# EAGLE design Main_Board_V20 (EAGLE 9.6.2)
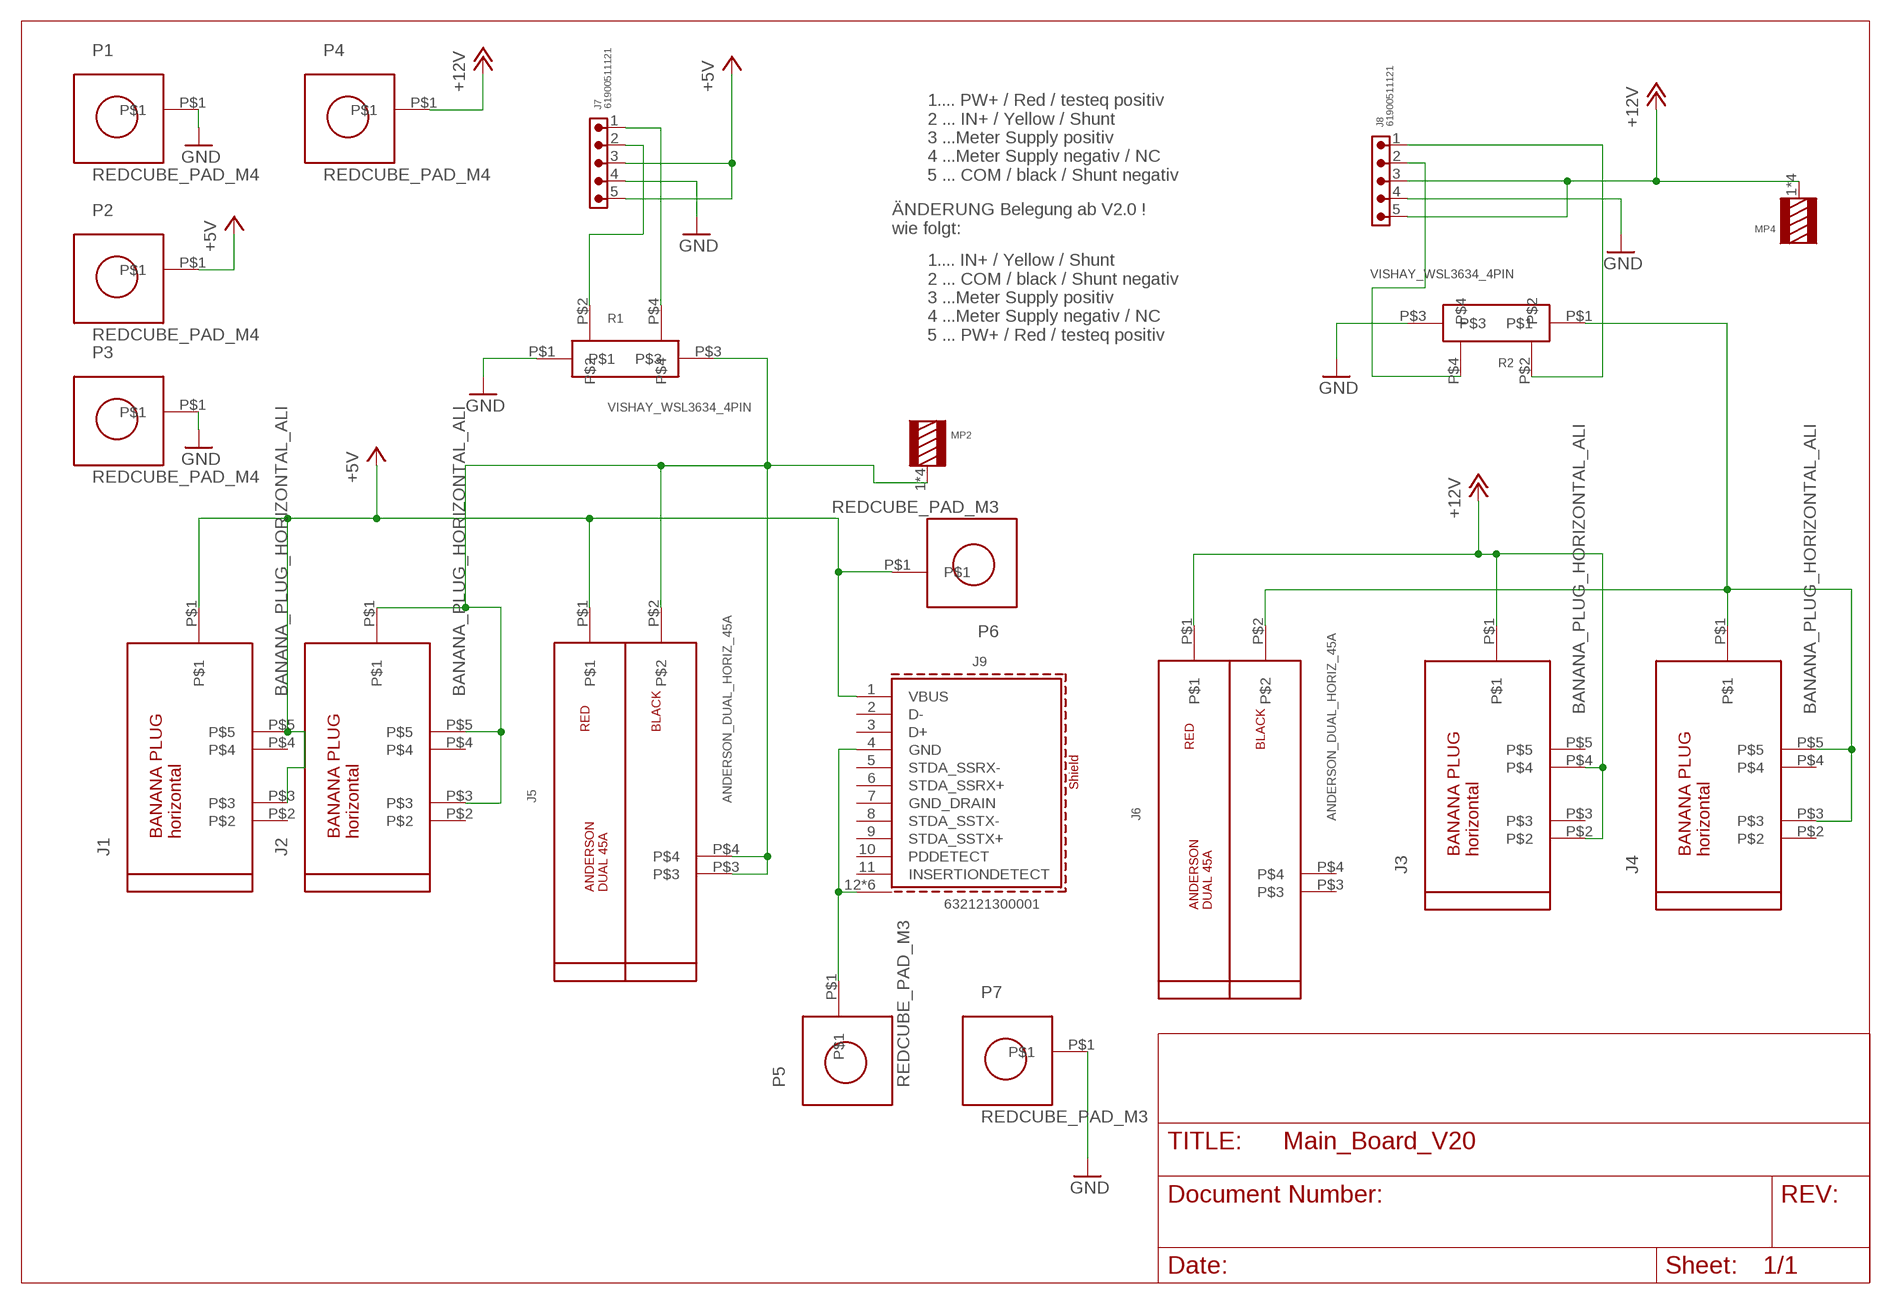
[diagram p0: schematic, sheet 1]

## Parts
J1  BANANA_PLUG_HORIZONTAL_ALI  [BANANA_PLUG_HORIZONTAL_ALI]
J2  BANANA_PLUG_HORIZONTAL_ALI  [BANANA_PLUG_HORIZONTAL_ALI]
J3  BANANA_PLUG_HORIZONTAL_ALI  [BANANA_PLUG_HORIZONTAL_ALI]
J4  BANANA_PLUG_HORIZONTAL_ALI  [BANANA_PLUG_HORIZONTAL_ALI]
J5  ANDERSON_DUAL_HORIZ_45A  [ANDERSON_DUAL_HORIZ_45A]
J6  ANDERSON_DUAL_HORIZ_45A  [ANDERSON_DUAL_HORIZ_45A]
J7  61900511121  61900511121  [61900511121]
J8  61900511121  61900511121  [61900511121]
J9  632121300001  [632121300001_MILLING_LINES]
MP2  WP-THRBU_THROUGH-HOLE_74650073R  [WP-THRBU_74650073]
MP4  WP-THRBU_THROUGH-HOLE_74650073R  [WP-THRBU_74650073]
P1  REDCUBE_PAD_M4  [REDCUBE_PAD_M4]
P2  REDCUBE_PAD_M4  [REDCUBE_PAD_M4]
P3  REDCUBE_PAD_M4  [REDCUBE_PAD_M4]
P4  REDCUBE_PAD_M4  [REDCUBE_PAD_M4]
P5  REDCUBE_PAD_M3  [REDCUBE_PAD_M3]
P6  REDCUBE_PAD_M3  [REDCUBE_PAD_M3]
P7  REDCUBE_PAD_M3  [REDCUBE_PAD_M3]
R1  VISHAY_WSL3634_4PIN  [VISHAY_WSL3637_4PIN]
R2  VISHAY_WSL3634_4PIN  [VISHAY_WSL3637_4PIN]

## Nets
+5V [Versorgung]: J1.P$1 J1.P$3 J1.P$5 J5.P$1 J7.3 J7.5 J9.1(VBUS) P2.P$1 P6.P$1
+12V [Versorgung]: J3.P$1 J3.P$2 J3.P$4 J6.P$1 J8.3 J8.5 MP4.1 MP4.2 MP4.3 MP4.4 P4.P$1
GND [Versorgung]: J7.4 J8.4 P1.P$1 P3.P$1 P7.P$1 R1.P$1 R2.P$3
N$2 [Versorgung]: J4.P$1 J4.P$3 J4.P$5 J6.P$2 R2.P$1
N$3 [Versorgung]: J2.P$1 J2.P$3 J2.P$5 J5.P$2 J5.P$3 J5.P$4 MP2.1 MP2.2 MP2.3 MP2.4 R1.P$3
N$4: J8.1 R2.P$2
N$5: J8.2 R2.P$4
N$6: J7.1 R1.P$4
N$7 [Versorgung]: J9.4(GND) J9.12(SHIELD) J9.13(SHIELD) J9.S1(SHIELD) J9.S2(SHIELD) J9.S3(SHIELD) J9.S4(SHIELD) P5.P$1
N$8: J7.2 R1.P$2
Unconnected: J1.P$2 J1.P$4 J2.P$2 J2.P$4 J3.P$3 J3.P$5 J4.P$2 J4.P$4 J6.P$3 J6.P$4 J9.2(D-) J9.3(D+) J9.5(STDA_SSRX-) J9.6(STDA_SSRX+) J9.7(GND_DRAIN) J9.8(STDA_SSTX-) J9.9(STDA_SSTX+) J9.10(PDDETECT) J9.11(INSERTIONDETECT)

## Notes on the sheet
- 1.... PW+ / Red / testeq positiv
  2 ... IN+ / Yellow / Shunt
  3 ...Meter Supply positiv
  4 ...Meter Supply negativ / NC
  5 ... COM / black / Shunt negativ
- ÄNDERUNG Belegung ab V2.0 !
  wie folgt:
- 1.... IN+ / Yellow / Shunt
  2 ... COM / black / Shunt negativ
  3 ...Meter Supply positiv
  4 ...Meter Supply negativ / NC
  5 ... PW+ / Red / testeq positiv

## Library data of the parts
J1-J4 = Antec-Hood:BANANA_PLUG_HORIZONTAL_ALI
J5 J6 = Antec-Hood:ANDERSON_DUAL_HORIZ_45A
J7 J8 = Eagle_WR-WTB (rev20a):61900511121: WR-WTB 2.54 mm Male Locking Header KIND PROPERTIES: Pitch:2.54 mm Gender:Male MATERIAL PROPERTIES: Insulator Material :PA66 Insulator Flammability Rating:UL94 V-0 Insulator Color:Beige Contact Material:Copper Alloy Contact Plating:Tin Contact Type:Stamped GENERAL INFORMATION Operating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; CONTACT-RESISTANCE: 20mOhm; DATASHEET-URL: https://www.we-online.com/catalog/datasheet/61900511121.pdf; GENDER: Male; L: 12.7mm; MOUNT: THT; PACKAGING: Bag; PART-NUMBER: 61900511121; PCB-CABLE-PANEL: PCB; PINS: 5; PITCH: 2.54mm; TOL-R: max.; TYPE: Vertical; USE-WITH: WR-WTB 2.54 mm Female Terminal Housing; WORKING-VOLTAGE: 250V(AC)
J9 = Antec-Hood:632121300001: WR-COM USB 3.1 Type C Plug Horizontal 0.8 mm Kind Properties Durability:5 000 Mating cycles Quality Class:5 000 Mating cycles Connector Type:USB Gender:Receptacle Type:Horizontal General Information Operating Temperature:-20up to +85 °C Compliance:RoHS Electrical Properties IR 1:5A Working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; APPLICATION: USB 3.1; DATASHEET-URL: https://www.we-online.com/catalog/datasheet/632121300001.pdf; GERDER: Receptacle; INTERFACE-TYPE: Type A; IR1: 5A; MOUNT: THR; PACKAGING: Tray; PART-NUMBER: 632121300001; PINS: 9; TYPE: Horizontal; WORKING-VOLTAGE: 20V(DC)
MP2 MP4 = Eagle_WP-THRBU (rev19a):WP-THRBU_THROUGH-HOLE: WP-THRBU REDCUBE THR internal through-hole thread; DATASHEET-URL: https://katalog.we-online.de/em/datasheet/74650073R.pdf; IR: 50A; PART-NUMBER: 74650073R; PINS: 4; THREAD: M3
P1-P4 = Antec-Hood:REDCUBE_PAD_M4
P5-P7 = Antec-Hood:REDCUBE_PAD_M3
R1 R2 = Antec-Hood:VISHAY_WSL3634_4PIN

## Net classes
1 Versorgung: width 1 mm, drill 0.5 mm, clearance 1 mm

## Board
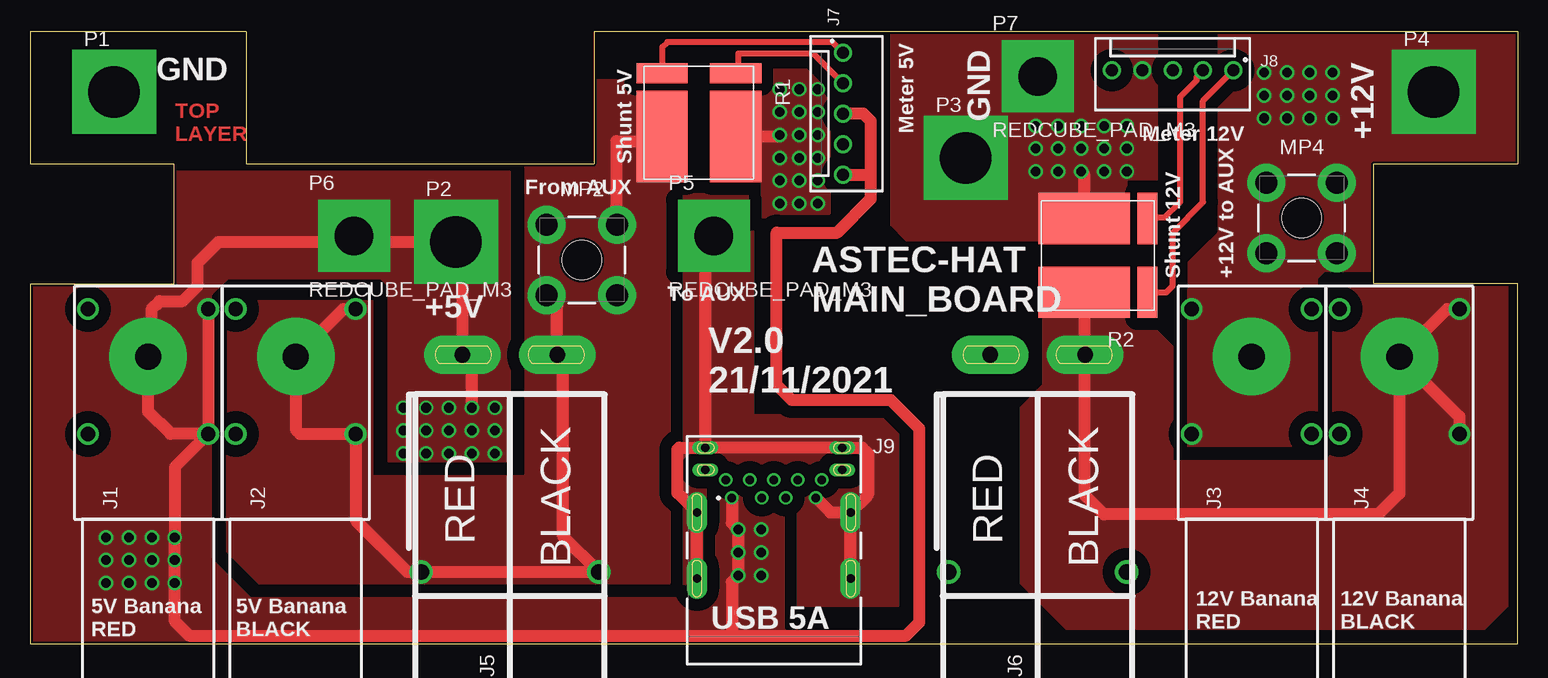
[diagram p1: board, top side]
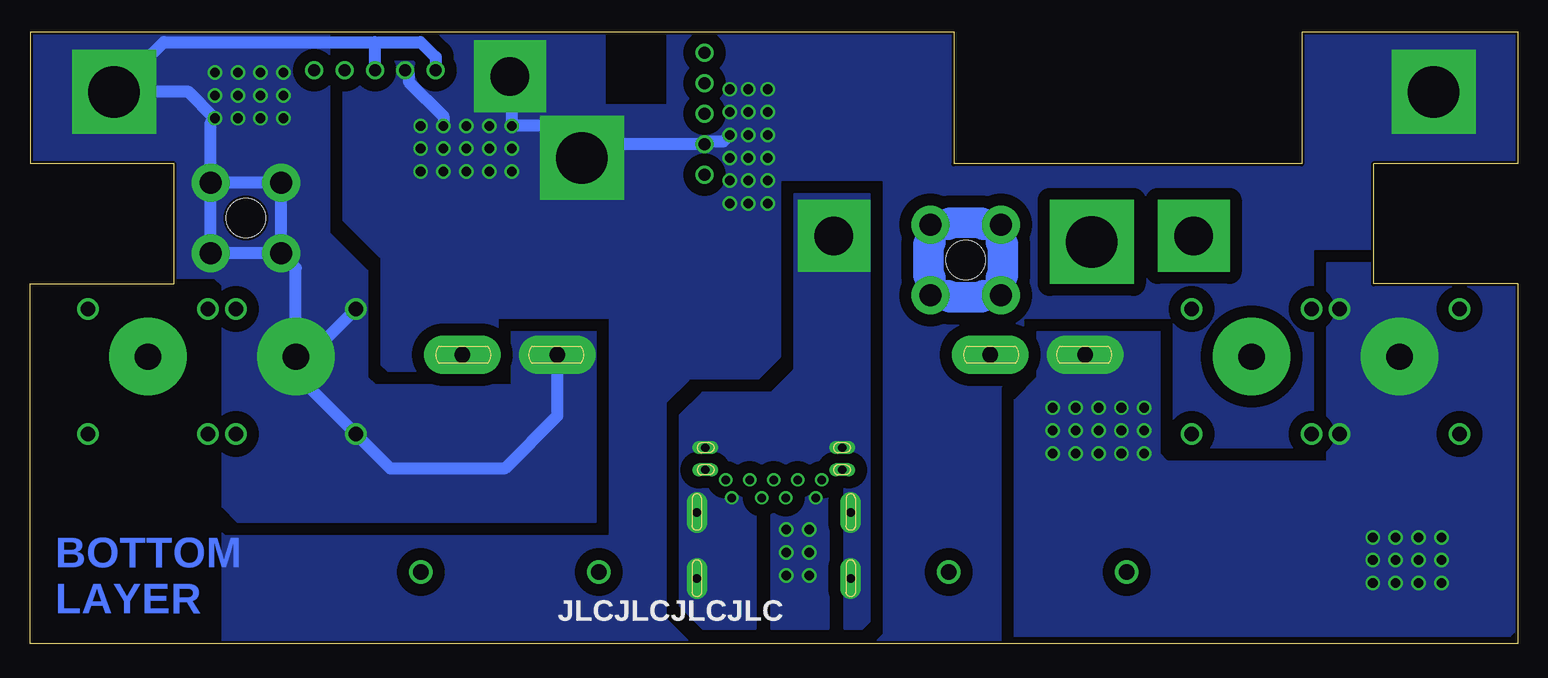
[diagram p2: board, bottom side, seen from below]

Size 124 x 51 mm. Coordinates in mm from the lower left corner, seen from the top.
Outline: 0,0 124,0 124,30 112,30 112,40 124,40 124,51 47,51 47,40 18,40 18,51 0,51 0,40 12,40 12,30 0,30 0,0
Copper layers (1*16): Top 0.035mm / dielectric 1.5mm / Bottom 0.035mm
Design rules "JLCPCB_2alyer": minimum track width 5mil, minimum drill 0.2mm, track to track 5mil, track to pad 0.2mm, pad to pad 0.2mm, via to via 0.2mm, smd to smd 5mil, copper to edge 0.2mm, drill to drill 0.5mm, minimum pad ring 0.13mm, minimum via ring 0.13mm, stop-mask expansion 0.05mm, vias tented up to drill 0mil, thermal gap 10mil
bRestrict: area 71,45 to 76,51

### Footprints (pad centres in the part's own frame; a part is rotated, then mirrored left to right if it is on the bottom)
BANANA_PLUG_HORIZONTAL_ALI = drill 2.2 pad 6.452: P$1 27.94,0 | drill 1.2: P$2 21.5,5; P$3 21.5,-5; P$4 31.9,5; P$5 31.9,-5
ANDERSON_DUAL_HORIZ_45A = drill 1.3 pad 3.2 long: P$1 28.1,3.95; P$2 28.1,-3.95 | drill 1.3: P$3 10,7.4; P$4 10,-7.4
61900511121 = drill 1: 1 5.08,0.3; 2 2.54,0.3; 3 0,0.3; 4 -2.54,0.3; 5 -5.08,0.3
632121300001_MILLING_LINES = drill 0.7 pad 1.1: 1 -3.5,4.425; 2 -1,4.425; 3 1,4.425; 4 3.5,4.425; 5 4,5.925; 6 2,5.925; 7 0,5.925; 8 -2,5.925; 9 -4,5.925 | drill 0.7 pad 1.1 long: 10 -5.7,6.765; 11 5.7,6.765; 12 5.7,8.605; 13 -5.7,8.605 | drill 0.7 pad 1.7 long: S1 -6.4,3.215; S2 6.4,3.215; S3 -6.4,-2.285; S4 6.4,-2.285
WP-THRBU_74650073 = drill 1.85 pad 3.2: 1 -2.935,-2.935; 2 -2.935,2.935; 3 2.935,2.935; 4 2.935,-2.935 | hole 3.3: 0,0
REDCUBE_PAD_M4 = drill 4.3 pad 7 square: P$1 0,0
REDCUBE_PAD_M3 = drill 3.2 pad 6 square: P$1 0,0
VISHAY_WSL3637_4PIN = smd 7.62 x 4.27: P$1 6.1,3.075; P$3 6.1,-3.075 | smd 1.68 x 4.27: P$2 0.84,3.075; P$4 0.84,-3.075

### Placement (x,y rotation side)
J1  9.85,-4 90 top
J2  22.15,-4 90 top
J3  101.85,-4 90 top
J4  114.15,-4 90 top
J5  40,-4 90 top
J6  84,-4 90 top
J7  68.07,44.2 90 top
J8  95.25,47.5 0 top
J9  62,7.75 0 top
MP2  46,32 0 top
MP4  106,35.5 0 top
P1  7,46 0 top
P2  35.5,33.5 0 top
P3  78,40.5 0 top
P4  117,46 0 top
P5  57,34 0 top
P6  27,34 0 top
P7  84,47.3 0 top
R1  55.75,48.39 270 top
R2  93.98,32.38 180 top

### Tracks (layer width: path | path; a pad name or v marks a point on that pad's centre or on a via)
+5V  (via drill 0.8)
  Top 1: 27.3,33.5 15.72,33.5 13.97,31.75 13.97,29.83 12.72,28.57 10.79,28.57 10.16,27.94 10.16,24.25 J1.P$1 9.85,19.36 11.71,17.5 J1.P$3 | 27.3,33.5 P2.P$1 36.05,32.95 J5.P$1 36.83,23.32 v36.83,19.68 | J7.3 69.47,44.2 70.1,43.56 70.1,38.99 | J7.5 69.98,39.12 70.1,38.99 | J1.P$3 12.06,14.71 v12.06,8.89 v12.06,6.99 v12.06,5.08 12.06,1.91 13.27,0.7 58.42,0.7 | J9.1 58.5,10.08 v59.05,9.53 v59.05,7.62 v59.05,5.71 58.5,5.16 58.5,0.78 58.42,0.7 | J1.P$5 J1.P$3 | 58.42,0.7 73.03,0.7 74.12,1.8 74.12,17.95 71.75,20.32 63.5,20.32 62.23,21.59 62.23,34.29 67.31,34.29 70.1,37.08 70.1,38.99 | P6.P$1 27.3,33.96 27.3,33.5
  other vias: 33.02,19.68 34.92,19.68 38.73,19.68 38.73,17.78 36.83,17.78 34.92,17.78 33.02,17.78 33.02,15.88 34.92,15.88 36.83,15.88 38.73,15.88 6.35,8.89 8.26,8.89 10.16,8.89 10.16,6.99 8.26,6.99 6.35,6.99 6.35,5.08 8.26,5.08 10.16,5.08 31.11,19.68 31.11,17.78 31.11,15.88 60.96,9.53 60.96,7.62 60.96,5.71
  pour Top (no thermals): 40.01,39.37 -0.64,39.37 -0.64,-0.64 -1.27,-1.27 65.41,-1.27 62.23,1.91 62.23,3.81 18.41,3.81 15.11,7.11 15.11,29.08 16.51,30.48 29.21,30.48 29.84,29.84 29.84,15.24 40.01,15.24
  pour Bottom (no thermals): 29.84,26.04 29.84,15.88 29.21,15.24 17.14,15.24 15.88,15.24 15.88,31.75 -1.27,31.75 -1.91,31.11 -1.91,3.17 0,1.27 0.64,0.64 41.91,0.64 41.91,19.05 41.91,20.32 40.01,22.23 40.01,26.04
  pour Top (no thermals): 56.52,13.34 56.52,0.64 62.87,0.64 62.87,13.34
  pour Bottom (no thermals): 62.23,13.34 62.23,1.27 57.4,1.27 57.4,13.34
+12V  (via drill 0.8)
  Bottom 1: J3.P$1 100.81,23.94 J3.P$4 | J6.P$1 80.05,19.01 84.45,14.61 93.95,14.61 J3.P$2 101.85,22.5 J3.P$1 | P4.P$1 110.77,46 v108.58,43.81 108.94,43.47 MP4.3 | 113.52,49.48 P4.P$1 | MP4.1 101.85,31.35 J3.P$1 | MP4.1 MP4.4 MP4.3 | MP4.1 MP4.2 MP4.3 | 95.25,50.16 112.83,50.16 P4.P$1 | 95.25,50.16 91.44,50.16 90.17,48.9 J8.5 | J8.3 95.25,50.16
  other vias: 102.87,47.62 102.87,45.72 102.87,43.81 104.78,43.81 104.78,45.72 104.78,47.62 106.68,47.62 106.68,45.72 106.68,43.81 108.58,45.72 108.58,47.62
  pour Bottom (no thermals): 99.06,51.44 99.06,34.29 95.89,31.11 95.89,22.23 95.25,21.59 83.82,21.59 83.82,26.04 76.83,26.04 76.83,10.16 106.68,10.16 107.95,11.43 107.95,29.84 108.58,30.48 112.39,30.48 120.65,38.73 125.73,38.73 125.73,51.44
  pour Top (no thermals): 99.06,51.44 99.06,34.29 97.79,33.02 96.52,31.75 96.52,29.84 96.52,16.51 107.31,16.51 107.31,30.48 107.95,31.11 110.49,31.11 113.03,31.11 126.36,31.11 126.36,51.44
GND  (via drill 0.8)
  Top 1: v62.48,42.42 62.35,42.29 R1.P$1 | v87.63,39.37 87.88,39.12 R2.P$3
  Bottom 1: J8.4 92.42,47.51 92.42,46.87 89.53,43.98 v89.53,43.18 | v65.66,42.42 66.2,41.87 67.55,41.87 J7.4 76.84,41.66 P3.P$1 80.68,43.18 v83.82,43.18 83.82,47.12 P7.P$1
  other vias: 62.48,46.23 62.48,44.32 62.48,40.51 65.66,40.51 65.66,44.32 65.66,46.23 64.14,46.23 64.14,44.32 64.14,42.42 64.14,40.51 91.44,39.37 91.44,41.27 91.44,43.18 89.53,39.37 83.82,39.37 85.72,43.18 85.72,39.37 87.63,41.27 85.72,41.27 83.82,41.27 62.48,38.61 65.66,38.61 64.14,38.61 89.53,41.27 87.63,43.18 62.48,36.7 64.14,36.7 65.66,36.7
  pour Top (no thermals): 60.96,48.9 60.96,35.56 66.67,35.56 66.67,48.9
  pour Bottom (rank 2, no thermals): -1.27,53.34 -1.27,-7.62 0.64,-9.53 107.95,-9.53 107.95,55.24 0.64,55.24
  pour Top (no thermals): 71.75,50.8 71.75,34.92 73.03,33.66 91.44,33.66 91.44,38.73 93.98,38.73 93.98,50.8
N$2
  Top 1: J4.P$1 114.15,12.55 112.39,10.79 89.53,10.79 87.95,12.38 J6.P$2 87.95,29.24 R2.P$1 | J4.P$1 119.15,18.94 J4.P$3 | J4.P$1 118.11,27.9 J4.P$5
  pour Top (no thermals): 108.58,29.84 108.58,15.88 107.95,15.24 95.25,15.24 95.25,24.77 92.71,27.3 84.45,27.3 84.45,21.59 82.55,19.68 82.55,5.08 86.36,1.27 121.28,1.27 123.19,3.17 123.19,29.84
N$3
  Top 1: MP2.1 43.95,28.18 J5.P$2 44.45,23.6 44.45,8.95 J5.P$4 J5.P$3 31.46,6 27.15,10.31 J2.P$3 22.5,17.5 22.15,17.86 J2.P$1 26.11,27.9 J2.P$5 | 52.29,42.67 R1.P$3 | MP2.3 48.9,34.98 48.9,41.91 52.7,41.91
  Bottom 2.54: MP2.2 43.06,33.48 42.88,33.29 42.88,30.71 43.06,30.52 MP2.1 44.52,29.07 44.71,28.88 47.29,28.88 47.48,29.07 MP2.4 48.94,30.52 49.12,30.71 49.12,33.29 48.94,33.48 MP2.3 47.48,34.94 47.29,35.12 44.71,35.12 44.52,34.94 MP2.2
  pour Top (no thermals): 16.38,28.57 16.38,7.75 19.05,5.08 53.34,5.08 53.34,44.01 50.36,46.99 46.35,46.99 41.27,41.91 41.27,13.97 28.57,13.97 28.57,28.57
N$4
  Top 0.508: R2.P$2 94.72,29.31 95.25,29.84 95.25,34.29 97.79,36.83 97.79,45.26 J8.1
N$5
  Top 0.508: R2.P$4 93.24,35.56 94.61,35.56 95.89,36.83 95.89,45.6 97.25,46.97 97.25,47.26 J8.2
N$6
  Top 0.508: R1.P$4 52.7,47.57 52.7,49.73 53.14,50.16 66.88,50.16 J7.1
N$7
  Top 1: J9.S3 J9.S1 53.98,12.59 53.98,16.2 54.13,16.36 J9.13 | J9.S4 J9.S2 | J9.4 66.71,10.96 J9.S2 | J9.S2 69.85,12.41 69.85,15.88 69.37,16.36 J9.12 J9.13 | J9.13 56.3,33.3 P5.P$1
  Bottom 1: J9.S2 68.4,11.25
  pour Top (rank 2, no thermals): 53.98,37.47 53.98,3.17 72.39,3.17 72.39,17.78 71.12,19.05 60.33,19.05 60.33,37.47
  pour Bottom (no thermals): 60.33,37.47 60.33,22.86 62.23,20.95 67.94,20.95 69.85,19.05 69.85,3.17 67.94,1.27 63.5,1.27 63.5,13.97 62.87,14.61 56.52,14.61 56.13,14.22 56.13,1.27 54.61,1.27 53.98,1.91 53.98,37.47
N$8
  Top 0.508: 59.05,47.77 59.05,49.23 65.28,49.23 J7.2
  Top 1: R1.P$2 59.05,47.77

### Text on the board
Top: TOP / LAYER
Bottom: BOTTOM / LAYER
tPlace: GND | GND | Meter 5V | Meter 12V | +12V | Shunt 5V | From AUX | Shunt 12V | To AUX | +12V to AUX | ASTEC-HAT / MAIN_BOARD | +5V | V2.0 / 21/11/2021 | USB 5A | 5V Banana / RED | 5V Banana / BLACK | 12V Banana / RED | 12V Banana / BLACK
bPlace: JLCJLCJLCJLC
